// Version 2.0, 05.09.99: Änderungen:
// ASS-Flankenwechsel entfällt, löschen der ASS und int. Variablen bei Neustart
// ASS-Schnittstelle benötigt keinen Flankenwechsel 0->1. Auftrag wird im
// nächsten PLC-Zyklus nach Auftragsende ausgeführt.
// Netzwerk 'Auswertung Status FC8' wurde geändert.
// DBInstanz.DBD0 (ASS_neu) und interne Variablen bei Neustart(DB8.DBX45.0=1)gelöscht.
// Anwender-Programmierung im OB100 entfällt.
// Version 1.3, 21.04.97: Änderung:
// ASS23 'Abbruch Positionieren' neu, SS 22 Status von 1 nach 5 geändert
// Version 1.2, 12.08.96: Änderungen zu Version 1.1:
// Einfügung von Istpositions-Schnittstellen  im Instanz-DB für Wechselpositionen;
// Neue Belegung der Varaiblen im Instanz-DB durch diese Änderung.
// Version 1.1, 14.03.96: Änderungen zu Version 1.0:
// Erweiterung FB 90 auf 2 Spindeln:
// Änderung der Variablen NewToolMag_Wechsel in NewToolMag_Wechsel_S1
// usw. und Einführung neuer Variablen NewToolMag_Wechsel_S2 usw. für
// Spindel 2.
// Dadurch Verschiebung der int. Variblen von DIB 28 nach DIB 36.
// Änderung in OB100 mit Einsatz FB 90 Version 2.0 notwendig.
// Datei:QUIT_5

FUNCTION_BLOCK FB 90
TITLE = QUIT_WZV
VERSION : 2.0

Var
  ASS_neu: DINT ;	// Anwenderschnittstelle
  Fehler: BOOL;		// Fehlerbit
  FehlerNr : INT ;	// Error von FC8 gespeichert
  Reserve1: INT ;	// Reservewort 1
  IstPosWechselstMag1: INT ; // Magazin-Istposition Wechselstelle Mag 1
  IstPosWechselstMag2: INT ; // Magazin-Istposition Wechselstelle Mag 2
  IstPosWechselstGr1: INT ; // Magazin-Istposition Wechselstelle Greifer 1
  IstPosWechselstGr2: INT ; // Magazin-Istposition Wechselstelle Greifer 2
  Reserve2: INT ; 	// Reservewort 2
  TaskIdent : BYTE ;	// TaskIdent an FC8
  TaskIdentNo : BYTE ;	// TaskIdentNo an FC8
  NewToolMag : INT ;	// NewToolMag an FC8
  NewToolLoc : INT ;	// NewToolLoc an FC8
  OldToolMag : INT ;	// OldToolMag an FC8
  OldToolLoc : INT ;	// OldToolLoc an FC8
  Status : INT ;	// Status von FC8
  NewToolMag_Wechsel_S1 : INT ;	// NewToolMag im Wechsel Spindel 1
  NewToolLoc_Wechsel_S1 : INT ;	// NewToolLoc im Wechsel Spindel 1
  OldToolMag_Wechsel_S1 : INT ;	// OldToolMag im Wechsel Spindel 1
  OldToolLoc_Wechsel_S1 : INT ;	// OldToolLoc im Wechsel Spindel 1
  NewToolMag_Wechsel_S2 : INT ;	// NewToolMag im Wechsel Spindel 2
  NewToolLoc_Wechsel_S2 : INT ;	// NewToolLoc im Wechsel Spindel 2
  OldToolMag_Wechsel_S2 : INT ;	// OldToolMag im Wechsel Spindel 2
  OldToolLoc_Wechsel_S2 : INT ;	// OldToolLoc im Wechsel Spindel 2
  ASS_alt: DINT ;	// Anwenderschnittst. Altwert
  ASS_Aenderung: DINT ;	// Änderung ASS
  ASS_aktiv: DINT ;	// Anwenderschnittstelle aktiv
  Start : BOOL ;	// Start an FC8
  Ready : BOOL ;	// Ready von FC8
  Error : INT ;		// Error von FC8
  SchrittNr : BYTE ;	// Schrittnummer Sprungverteiler
END_VAR

VAR_TEMP
  ASS_TEMP : DINT ;	// Anwenderschnittstelle temporär
END_VAR

BEGIN
NETWORK
TITLE =Flankenauswertung

	UN    DB8.DBX 45.0;
	SPB   ANF; // Neustart ? ->
	L	0;
	T 	ASS_neu;
	T     ASS_alt;	// Anwenderschnittst. Altwert
	T	ASS_Aenderung; // Änderung ASS
  	T	ASS_aktiv; // Anwenderschnittstelle aktiv
  	R	Start; // Start an FC8
  	R	Ready; // Ready von FC8
	R	Fehler;
	BEA;
ANF:  L     ASS_neu; // Anwenderschnittstelle
      L     ASS_alt; // Altwert ASS
      XOD   ; // Flanke
      L     ASS_neu;
      T     ASS_alt;
      UD    ;
      L     ASS_Aenderung; // Änderung
      OD    ;
      T     ASS_Aenderung; // Alle Änderungen
      U     Start; // Start FC8
      SPB   FC8; // FC 8 aktiv ? Ja ->
      L     0;
      ==D   ;
      O     Fehler; // Fehler ? Ja -> Abbruch
      SPB   ENDE; // Änderung ? Nein -> Abbruch
NETWORK
TITLE =Sprungverteiler

      L     ASS_Aenderung; // Änderungen
      T     #ASS_TEMP;
      L     0;
      T     SchrittNr; // Schritt-Nr. auf 0
      L     1;
      T     ASS_aktiv; // Aktive Bitleiste auf 1
LOOP: L     #ASS_TEMP;
      SRD   1;
      SPP   SPL; // Sprung wenn geschobenes Bit = 1
      T     #ASS_TEMP;
      L     ASS_aktiv;
      SLD   1; // Aktive Bitleiste nachführen
      T     ASS_aktiv;
      L     SchrittNr;
      INC   1; // Schritt-Nr. + 1
      T     SchrittNr;
      L     32;
      >I    ;
      SPB   ENDE; // Schritt-Nr. > 32? Abbruch ->
      SPA   LOOP;
SPL:  L     SchrittNr;
      SPL   END1;
      SPA   SS25;
      SPA   SS26;
      SPA   SS27;
      SPA   SS28;
      SPA   SS29;
      SPA   SS30;
      SPA   SS31;
      SPA   SS32;
      SPA   SS17;
      SPA   SS18;
      SPA   SS19;
      SPA   SS20;
      SPA   SS21;
      SPA   SS22;
      SPA   SS23;
      SPA   SS24;
      SPA   SS9;
      SPA   SS10;
      SPA   SS11;
      SPA   SS12;
      SPA   SS13;
      SPA   SS14;
      SPA   SS15;
      SPA   SS16;
      SPA   SS1;
      SPA   SS2;
      SPA   SS3;
      SPA   SS4;
      SPA   SS5;
      SPA   SS6;
      SPA   SS7;
      SPA   SS8;
END1: SPA   ENDE;
NETWORK
TITLE =SS1,SS2: Quittung WKZ-Beladen und Reset WKZ-Beladen

SS2:  L     3; // Status = 3 bei Reset
      SPA   STA1;
SS1:  L     1; // Status = 1 bei beendet
STA1: T     Status;
      L     1;
      T     TaskIdent;
      L     3;
      T     TaskIdentNo; // TaskIdentNo = 3 Beladestelle Magazin
      L     DB71.DBW   88; // Magazin-Nr. Beladen
      T     NewToolMag;
      L     DB71.DBW   90; // Platz.-Nr. Beladen
      T     NewToolLoc;
      L     0;
      T     OldToolMag;
      T     OldToolLoc;
      SPA   FC8S;
NETWORK
TITLE =SS3,SS4: Quittung WKZ-Entladen und Reset WKZ-Entladen

SS4:  L     3; // Status = 3 bei Reset
      SPA   STA3;
SS3:  L     1; // Status = 1 bei beendet
STA3: T     Status;
      L     1;
      T     TaskIdent;
      L     3;
      T     TaskIdentNo; // TaskIdentNo = 3 Beladestelle Magazin
      L     0;
      T     NewToolMag;
      T     NewToolLoc;
      L     DB71.DBW   80; // Magazin-Nr. Entladen
      T     OldToolMag;
      L     DB71.DBW   82; // Platz-Nr. Entladen
      T     OldToolLoc;
      SPA   FC8S;
NETWORK
TITLE =SS5,SS6:Quittung Wechsel vorber.Spi1,Reset Wechsel vorber.Spi1

SS6:  L     3; // Status = 3 bei Reset
      SPA   STA5;
SS5:  L     1; // Status = 1 bei beendet
STA5: T     Status;
      L     2;
      T     TaskIdent; // TaskIdent = 2 (DB72)
      L     1;
      T     TaskIdentNo; // TaskIdentNo = 1 (SS 1)
      L     DB72.DBW   24; // Magazin-Nr. neues Werkzeug
      T     NewToolMag;
      T     NewToolMag_Wechsel_S1;
      L     DB72.DBW   26; // Platz-Nr. neues Werkzeug
      T     NewToolLoc;
      T     NewToolLoc_Wechsel_S1;
      L     DB72.DBW   30; // Platz-Nr. altes Werkzeug
      L     0;
      <>I   ;
      SPB   OLD1; // Werkzeug in Spindel ? ja ->
      T     OldToolMag;
      T     OldToolLoc;
      T     OldToolMag_Wechsel_S1;
      T     OldToolLoc_Wechsel_S1;
      SPA   FC8S;
OLD1: L     DB72.DBW   20; // Magazin-Nr. Spindel
      T     OldToolMag;
      T     OldToolMag_Wechsel_S1;
      L     DB72.DBW   22; // Platz-Nr. Spindel
      T     OldToolLoc;
      T     OldToolLoc_Wechsel_S1;
      SPA   FC8S;
NETWORK
TITLE =SS7,SS8:Quittg Wechsel vorber.Spi2,Reset Wechsel vorber.Spi2

SS8:  L     3; // Status = 3 bei Reset
      SPA   STA6;
SS7:  L     1; // Status = 1 bei beendet
STA6: T     Status;
      L     2;
      T     TaskIdent; // TaskIdent = 2 (DB72)
      L     2;
      T     TaskIdentNo; // TaskIdentNo = 2 (SS 2)
      L     DB72.DBW   72; // Magazin-Nr. neues Werkzeug
      T     NewToolMag;
      T     NewToolMag_Wechsel_S2;
      L     DB72.DBW   74; // Platz-Nr. neues Werkzeug
      T     NewToolLoc;
      T     NewToolLoc_Wechsel_S2;
      L     DB72.DBW   78; // Platz-Nr. altes Werkzeug
      L     0;
      <>I   ;
      SPB   OLD2; // Werkzeug in Spindel ? ja ->
      T     OldToolMag;
      T     OldToolLoc;
      T     OldToolMag_Wechsel_S2;
      T     OldToolLoc_Wechsel_S2;
      SPA   FC8S;
OLD2: L     DB72.DBW   68; // Magazin-Nr. Spindel
      T     OldToolMag;
      T     OldToolMag_Wechsel_S2;
      L     DB72.DBW   70; // Platz-Nr. Spindel
      T     OldToolLoc;
      T     OldToolLoc_Wechsel_S2;
      SPA   FC8S;
NETWORK
TITLE =SS9: Status-Änderung Spindel 1 -> Magazin

SS9:  L     1; // Status = 1 Wechsel beendet
      T     Status;
      L     2;
      T     TaskIdent; // TaskIdent = 2 (DB72)
      L     1;
      T     TaskIdentNo; // TaskIdentNo = 1 (SS 1)
      L     DB72.DBW   26; // Platz-Nr. neues Werkzeug
      L     0;
      <>I   ;
      SPB   NEW9; // TO programmiert ? Nein ->
      T     NewToolMag;
      T     NewToolLoc;
      T     NewToolMag_Wechsel_S1;
      T     NewToolLoc_Wechsel_S1;
      SPA   OLD9;
NEW9: L     105; // Status = 105 Wechsel läuft
      T     Status;
      L     DB72.DBW   24; // Quelle neues Werkzeug Magazin
      T     NewToolMag;
      T     NewToolMag_Wechsel_S1;
      L     DB72.DBW   26; // Quelle neues Werkzeug Platz
      T     NewToolLoc;
      T     NewToolLoc_Wechsel_S1;
OLD9: L     DB72.DBW   28; // Magazin-Nr. altes Werkzeug
      T     OldToolMag;
      T     OldToolMag_Wechsel_S1;
      L     DB72.DBW   30; // Platz-Nr. altes Werkzeug
      T     OldToolLoc;
      T     OldToolLoc_Wechsel_S1;
      SPA   FC8S;

NETWORK
TITLE =SS10: Status-Änderung Magazin -> Spindel 1

SS10: L     1; // Status = 1 Wechsel beendet
      T     Status;
      L     2;
      T     TaskIdent; // TaskIdent = 2 (DB72)
      L     1;
      T     TaskIdentNo; // TaskIdentNo = 1 (SS 1)
      L     DB72.DBW   20; // Zielposition neues Werkzeug Magazin
      T     NewToolMag;
      T     NewToolMag_Wechsel_S1;
      L     DB72.DBW   22; // Zielposition neues Werkzeug Platz
      T     NewToolLoc;
      T     NewToolLoc_Wechsel_S1;
      L     DB72.DBW   28; // Magazin-Nr. altes Werkzeug
      T     OldToolMag;
      T     OldToolMag_Wechsel_S1;
      L     DB72.DBW   30; // Platz-Nr. altes Werkzeug
      T     OldToolLoc;
      T     OldToolLoc_Wechsel_S1;
      SPA   FC8S;

NETWORK
TITLE =SS11: Abbruch/Reset Wechsel Spindel 1

SS11: L     3; // Status = 3 Abbruch Wechsel
      T     Status;
      L     2;
      T     TaskIdent; // TaskIdent = 2 (DB72)
      L     1;
      T     TaskIdentNo; // TaskIdentNo = 1 (SS 1)
      L     NewToolMag_Wechsel_S1;
      T     NewToolMag;
      L     NewToolLoc_Wechsel_S1;
      T     NewToolLoc;
      L     OldToolMag_Wechsel_S1;
      T     OldToolMag;
      L     OldToolLoc_Wechsel_S1;
      T     OldToolLoc;
      SPA   FC8S;
NETWORK
TITLE =SS12: Status-Änderung Spindel 2 -> Magazin

SS12: L     1; // Status = 1 Wechsel beendet
      T     Status;
      L     2;
      T     TaskIdent; // TaskIdent = 2 (DB72)
      L     2;
      T     TaskIdentNo; // TaskIdentNo = 2 (SS 2)
      L     DB72.DBW   74; // Platz-Nr. neues Werkzeug
      L     0;
      <>I   ;
      SPB   NE12; // TO programmiert ? Nein ->
      T     NewToolMag;
      T     NewToolLoc;
      T     NewToolMag_Wechsel_S2;
      T     NewToolLoc_Wechsel_S2;
      SPA   OL12;
NE12: L     105; // Status = 105 Wechsel läuft
      T     Status;
      L     DB72.DBW   72; // Quelle neues Werkzeug Magazin
      T     NewToolMag;
      T     NewToolMag_Wechsel_S2;
      L     DB72.DBW   74; // Quelle neues Werkzeug Platz
      T     NewToolLoc;
      T     NewToolLoc_Wechsel_S2;
OL12: L     DB72.DBW   76; // Magazin-Nr. altes Werkzeug
      T     OldToolMag;
      T     OldToolMag_Wechsel_S2;
      L     DB72.DBW   78; // Platz-Nr. altes Werkzeug
      T     OldToolLoc;
      T     OldToolLoc_Wechsel_S2;
      SPA   FC8S;

NETWORK
TITLE =SS13: Status-Änderung Magazin -> Spindel 2

SS13: L     1; // Status = 1 Wechsel beendet
      T     Status;
      L     2;
      T     TaskIdent; // TaskIdent = 2 (DB72)
      L     2;
      T     TaskIdentNo; // TaskIdentNo = 2 (SS 2)
      L     DB72.DBW   68; // Zielposition neues Werkzeug Magazin
      T     NewToolMag;
      T     NewToolMag_Wechsel_S2;
      L     DB72.DBW   70; // Zielposition neues Werkzeug Platz
      T     NewToolLoc;
      T     NewToolLoc_Wechsel_S2;
      L     DB72.DBW   76; // Magazin-Nr. altes Werkzeug
      T     OldToolMag;
      T     OldToolMag_Wechsel_S2;
      L     DB72.DBW   78; // Platz-Nr. altes Werkzeug
      T     OldToolLoc;
      T     OldToolLoc_Wechsel_S2;
      SPA   FC8S;

NETWORK
TITLE =SS14: Abbruch/Reset Wechsel Spindel 2

SS14: L     3; // Status = 3 Abbruch Wechsel
      T     Status;
      L     2;
      T     TaskIdent; // TaskIdent = 2 (DB72)
      L     2;
      T     TaskIdentNo; // TaskIdentNo = 2 (SS 2)
      L     NewToolMag_Wechsel_S2;
      T     NewToolMag;
      L     NewToolLoc_Wechsel_S2;
      T     NewToolLoc;
      L     OldToolMag_Wechsel_S2;
      T     OldToolMag;
      L     OldToolLoc_Wechsel_S2;
      T     OldToolLoc;
      SPA   FC8S;
NETWORK
TITLE =SS15: Quittung Umladen MMC

SS15: L     1; // Status = 1 Umladen beendet
      T     Status;
      L     1;
      T     TaskIdent; // TaskIdent = 1 (DB71)
      L     1;
      T     TaskIdentNo; // TaskIdentNo = 1
      L     DB71.DBW   28; // Magazin-Nr. Ziel Umladen
      T     NewToolMag;
      L     DB71.DBW   30; // Platz-Nr. Ziel Umladen
      T     NewToolLoc;
      L     0;
      T     OldToolMag;
      T     OldToolLoc;
      SPA   FC8S;
NETWORK
TITLE =SS16: Asynchrones umspeichern Spindel 1 -> Magazin

SS16: L     1; // Status = 1
      T     Status;
      L     4;
      T     TaskIdent; // TaskIdent = 4 (Auftrag von PLC)
      L     1;
      T     TaskIdentNo; // TaskIdentNo = 1 (Kanal 1)
      L     1; // Magazin-Nr. Ziel = 1
      T     NewToolMag;
      L     IstPosWechselstMag1; // Platz-Nr. Ziel = Istposition Magazin
      T     NewToolLoc;
      L     9998; // Magazin-Nr. Quelle = Zwischenspeicher
      T     OldToolMag;
      L     1; // Platz-Nr. Quelle = Spindel 1
      T     OldToolLoc;
      SPA   FC8S;
NETWORK
TITLE =SS17: Asynchrones umspeichern Magazin -> Spindel 1

SS17: L     1; // Status = 1
      T     Status;
      L     4;
      T     TaskIdent; // TaskIdent = 4 (Auftrag von PLC)
      L     1;
      T     TaskIdentNo; // TaskIdentNo = 1 (Kanal 1)
      L     9998; // Magazin-Nr. Ziel = Zwischenspeicher
      T     NewToolMag;
      L     1;	  // Platz-Nr. Ziel = Spindel 1
      T     NewToolLoc;
      L     1; // Magazin-Nr. Quelle = Magazin-Nr.
      T     OldToolMag;
      L     IstPosWechselstMag1; // Platz-Nr. Quelle = Istposition
      T     OldToolLoc;
      SPA   FC8S;
NETWORK
TITLE =SS18: Asynchrones umspeichern Spindel 2 -> Magazin

SS18: L     1; // Status = 1
      T     Status;
      L     4;
      T     TaskIdent; // TaskIdent = 4 (Auftrag von PLC)
      L     2;
      T     TaskIdentNo; // TaskIdentNo = 2 (Kanal 2)
      L     1; // Magazin-Nr. Ziel = 1
      T     NewToolMag;
      L     IstPosWechselstMag1; // Platz-Nr. Ziel = Istposition Magazin
      T     NewToolLoc;
      L     9998; // Magazin-Nr. Quelle = Zwischenspeicher
      T     OldToolMag;
      L     2; // Platz-Nr. Quelle = Spindel 2
      T     OldToolLoc;
      SPA   FC8S;
NETWORK
TITLE =SS19: Asynchrones umspeichern Magazin -> Spindel 2

SS19: L     1; // Status = 1
      T     Status;
      L     4;
      T     TaskIdent; // TaskIdent = 4 (Auftrag von PLC)
      L     2;
      T     TaskIdentNo; // TaskIdentNo = 2 (Kanal 2)
      L     9998; // Magazin-Nr. Ziel = Zwischenspeicher
      T     NewToolMag;
      L     2;	  // Platz-Nr. Ziel = Spindel 2
      T     NewToolLoc;
      L     1; // Magazin-Nr. Quelle = Magazin-Nr.
      T     OldToolMag;
      L     IstPosWechselstMag1; // Platz-Nr. Quelle = Istposition
      T     OldToolLoc;
      SPA   FC8S;
NETWORK
TITLE =SS20: Änderung Istposition

SS20: L     5; 	// Status = 5
      T     Status;
      L     4;
      T     TaskIdent; // TaskIdent = 4 (Auftrag von PLC)
      L     1;
      T     TaskIdentNo; // TaskIdentNo = 1 (Kanal 1)
      L     1; 	// Magazin-Nr. Ziel = 1
      T     NewToolMag;
      L     IstPosWechselstMag1; // Platz-Nr. Ziel = Istpos.Greifer 1
      T     NewToolLoc;
      L     9998; // Magazin-Nr. Quelle = Zwischenspeicher
      T     OldToolMag;
      L     1; // Platz-Nr. Quelle = Spindel
      T     OldToolLoc;
      SPA   FC8S;
NETWORK
TITLE =SS21:

SS21: SPA   LOE1;
NETWORK
TITLE =SS22/SS23: Quittung/Abbruch positionieren zur Beladestelle

SS23: L 3; 			// Status = 3 Abbruch
      SPA ST22;
SS22: L     5; 		// Status = 5
ST22: T     Status;
      L     1;
      T     TaskIdent; 	// TaskIdent = 1 (DB 71)
      L     3;
      T     TaskIdentNo;	// TaskIdentNo = 3 Beladestelle Magazin
      L     DB71.DBW 80; 	// Magazin-Nr. Ziel = Magazin-Nr. der Beladestelle
      T     NewToolMag;
      L     DB71.DBW 82; 	// Platz-Nr. Ziel = Platz-Nr. der Beladestelle
      T     NewToolLoc;
      L     0;
      T     OldToolMag;  	// Magazin-Nr. = 0
      T     OldToolLoc;	// Platz-Nr. = 0
      SPA   FC8S;
NETWORK
TITLE =SS24:

SS24: SPA   LOE1;
NETWORK
TITLE =SS25:

SS25: SPA   LOE1;
NETWORK
TITLE =SS26:

SS26: SPA   LOE1;
NETWORK
TITLE =SS27:

SS27: SPA   LOE1;
NETWORK
TITLE =SS28:

SS28: SPA   LOE1;
NETWORK
TITLE =SS29:

SS29: SPA   LOE1;
NETWORK
TITLE =SS30:

SS30: SPA   LOE1;
NETWORK
TITLE =SS31:

SS31: SPA   LOE1;
NETWORK
TITLE =SS32:

SS32: SPA   LOE1;
NETWORK
TITLE =Aufruf FC8

FC8S: SET   ;
      S     Start; //Start FC8
FC8:  CALL FC     8 (
           Start                    := Start,
           TaskIdent                := TaskIdent,
           TaskIdentNo              := TaskIdentNo,
           NewToolMag               := NewToolMag,
           NewToolLoc               := NewToolLoc,
           OldToolMag               := OldToolMag,
           OldToolLoc               := OldToolLoc,
           Status                   := Status,
           Ready                    := Ready,
           Error                    := Error);

NETWORK
TITLE =Auswertung Status FC8

      UN    Start;
      SPB   ENDE; // FC 8 aktiv ? Nein ->
      UN    Ready;
      SPB   ERRO; // Ready FC 8 = 1 ? Nein ->
      R     Start;
      SPA   LOE;
ERRO: L     0;
      L     Error; // Fehler-Wort
      ==I   ;
      SPB   ENDE; // Auftrag mit Fehler beendet
      T     FehlerNr; // Fehler-Nr. speichern
      R     Start;
      L Status;
      L 3;
      <>I;	// bei Status 3 kein Fehlerbit setzen
      S     Fehler;
LOE:  L     ASS_aktiv; // Aktivleiste
      INVD  ; // Invertieren
      L     ASS_neu; // Anwenderschnittstelle
      UD    ;
      T     ASS_neu; // Bearbeitetes Bit ASS löschen
LOE1: L     ASS_Aenderung; // Änderung
      L     ASS_aktiv;
      INVD  ;
      UD    ;
      T     ASS_Aenderung; //Bearbeitetes Änderungsbit löschen
	L     ASS_alt;
      L     ASS_aktiv;
      INVD  ;
      UD    ;
      T     ASS_alt; //Bearbeitetes Alt-SS löschen
ENDE: NOP   0;
END_FUNCTION_BlOCK

DATA_BLOCK db 90

        VERSION: 1.0

fb 90
Begin
END_DATA_BLOCK

